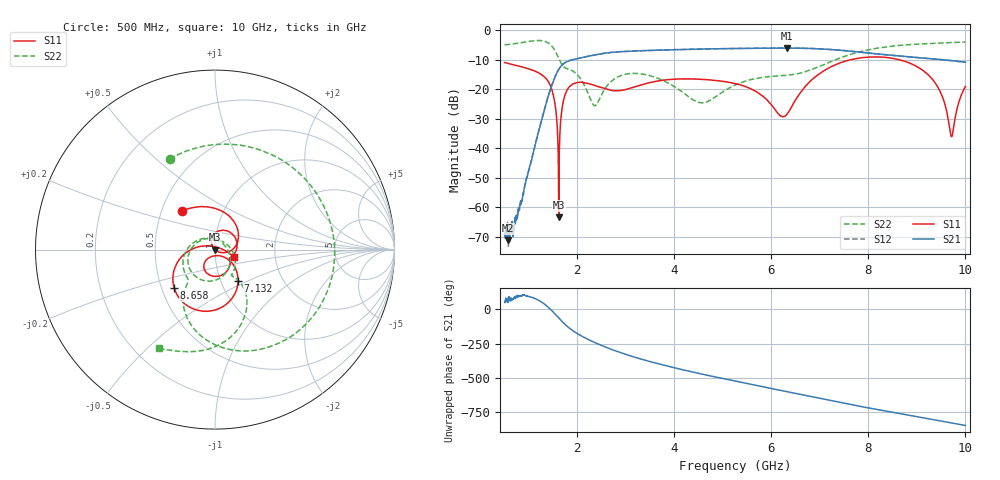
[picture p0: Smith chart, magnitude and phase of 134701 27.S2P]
!  2-Port S-parameters saved by WinCal
! VAR MeasName=S-Parameters (CALIBRATED_DATA) read from VNA (N5242A)
! VAR MeasDate=2013-7-3 16:32:47
! VAR NAME=134701 27
! VAR FILENAME=134701 27.S2P
! VAR DATE=2013-7-3 16:32:47
! VAR PHYS_PORTS=1,2
# Hz S MA R 50
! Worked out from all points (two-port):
!   1601 points, 500 MHz to 10 GHz, reference 50 ohm
!   highest |S21| = -6.07 dB at 6.325 GHz (marker M1); lowest = -71.2 dB at 571.2 MHz (marker M2)
!   |S21| within 3 dB of the highest: 2.155 GHz to 8.855 GHz (6.7 GHz wide, 122 % of centre)
!   lowest |S11| = -63.4 dB at 1.616 GHz (marker M3), VSWR 1.00, Z = 49.9 + j0.0447 ohm
!   |S11| at or under -10 dB: start of sweep to 7.637 GHz; 8.631 GHz to end of sweep
!   |S22| runs from -25.6 to -3.5 dB; largest |S21 - S12| = 0.003
!   S11 on the Smith chart (normalised r, x): 500 MHz: 0.64, +0.30; 7.132 GHz: 1.21, -0.44; 8.658 GHz: 0.58, -0.28; 10 GHz: 1.23, -0.10
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5e8  0.2825 130.1  0.000347 53.9  0.0003932 67.3  0.5644 116.6
5.7125e8  0.273 123.8  0.0002757 51.6  0.0004031 60.5  0.5717 106.4
8.8e8  0.2354 94.8  0.001746 103.0  0.001602 102.1  0.619 56.1
1.153125e9  0.1976 62.9  0.01353 75.3  0.0135 75.8  0.6671 -1.2
1.461875e9  0.1054 4.0  0.1097 -4.7  0.1096 -4.8  0.551 -84.8
1.61625e9  0.0006777 138.6  0.2168 -61.9  0.2164 -61.9  0.3329 -122.2
1.764688e9  0.08776 92.6  0.2877 -115.3  0.2876 -115.3  0.2256 -131.6
2.085312e9  0.1308 28.9  0.3418 166.4  0.342 166.5  0.1416 171.5
2.358438e9  0.1156 -5.0  0.3804 118.8  0.3807 118.8  0.05244 58.0
2.679062e9  0.09656 -26.7  0.4176 71.9  0.4182 71.9  0.1314 -56.2
3.154062e9  0.1077 -38.8  0.443 14.7  0.443 14.7  0.1853 -119.1
3.670625e9  0.1384 -62.1  0.4583 -36.2  0.4577 -36.2  0.1515 -167.8
4.549375e9  0.1468 -98.1  0.4781 -109.7  0.4788 -109.7  0.0589 75.9
5.25e9  0.1247 -118.7  0.4884 -162.6  0.489 -162.6  0.1171 -20.6
6.324688e9  0.03819 -62.8  0.4969 120.4  0.4966 120.3  0.1722 -57.4
6.835312e9  0.1443 -41.1  0.4882 83.4  0.4889 83.5  0.2156 -52.9
7.132188e9  0.2171 -53.8  0.4748 62.1  0.4758 62.0  0.2712 -53.4
8.420625e9  0.3405 -123.7  0.3785 -24.5  0.3779 -24.8  0.5277 -86.8
8.658125e9  0.3122 -136.8  0.3633 -39.4  0.3634 -39.6  0.5525 -93.2
9.370625e9  0.1296 179.1  0.3243 -84.6  0.3237 -84.8  0.5983 -108.7
9.715e9  0.01562 77.4  0.305 -107.1  0.3034 -107.2  0.6161 -114.8
1e10  0.1111 -21.5  0.2868 -125.5  0.2858 -125.7  0.6308 -119.4
